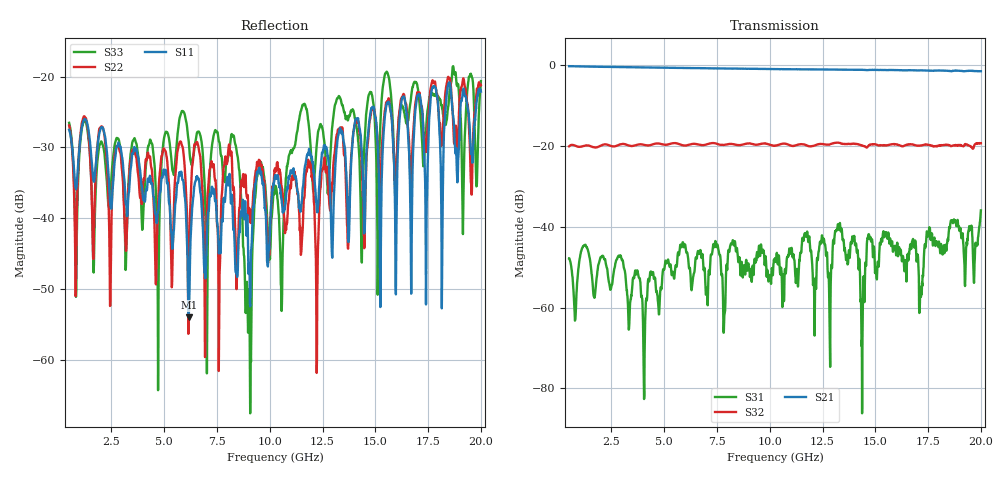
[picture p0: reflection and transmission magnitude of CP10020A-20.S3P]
!Agilent Technologies,E5071C,MY46316741,A.11.02
!Date: Thu Jan 10 14:58:44 2019
!Data & Calibration Information:
!Freq	S22:SOLT3(ON)	S23:SOLT3(ON)	S24:SOLT3(ON)
!	S32:SOLT3(ON)	S33:SOLT3(ON)	S34:SOLT3(ON)
!	S42:SOLT3(ON)	S43:SOLT3(ON)	S44:SOLT3(ON)
!PortZ  Port2:50+j0  Port3:50+j0  Port4:50+j0
!Above PortZ is port z conversion or system Z0 setting when saving the data.
!When reading, reference impedance value at option line is always used.
# Hz S dB R 50
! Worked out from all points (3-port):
!   1561 points, 500 MHz to 20 GHz, reference 50 ohm
!   strongest paths, dB at 500 MHz, 5.375 GHz, 10.25 GHz, 15.12 GHz, 20 GHz:
!     S21: -0.2, -0.6, -0.9, -1.1, -1.4
!     S32: -20.0, -19.3, -19.9, -19.8, -19.3
!     S31: -47.8, -51.9, -47.8, -48.7, -35.9
!   lowest |S11| = -54.0 dB at 6.162 GHz (marker M1), VSWR 1.00, Z = 49.8 + j0.0902 ohm
!   |S11| at or under -10 dB: start of sweep to end of sweep
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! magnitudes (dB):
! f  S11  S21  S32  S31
! 500 MHz  -27.5  -0.2  -20.0  -47.8
! 4.062 GHz  -37.0  -0.5  -19.7  -81.7
! 6.162 GHz  -54.0  -0.6  -19.7  -49.6
! 8.325 GHz  -42.6  -0.8  -19.6  -44.1
! 9.05 GHz  -48.1  -0.8  -19.3  -51.3
! 10.25 GHz  -34.0  -0.9  -19.9  -47.8
! 12.24 GHz  -39.1  -1.0  -19.6  -47.9
! 13.31 GHz  -27.4  -1.1  -19.2  -39.2
! 14.4 GHz  -32.9  -1.1  -19.9  -64.2
! 20 GHz  -22.1  -1.4  -19.3  -35.9
